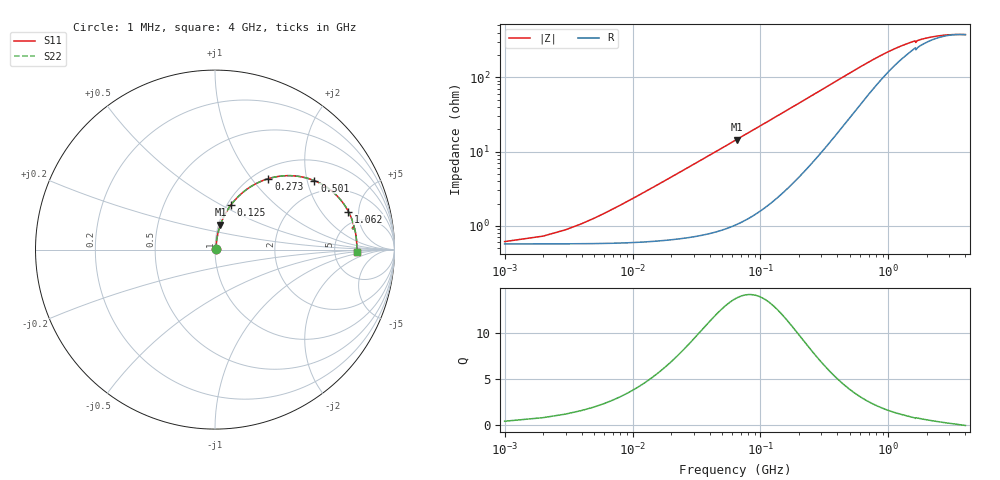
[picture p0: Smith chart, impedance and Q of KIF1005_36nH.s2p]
!version-2
!date-12.2020
!Series
# MHz S RI R 50
!Freq ReS11 ImS11 ReS21 ImS21 ReS12 ImS12 ReS22 ImS22
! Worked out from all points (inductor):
!   4000 points, 1 MHz to 4 GHz, reference 50 ohm
!   read as one part in series: L = 35.5 nH near 21 MHz
!   highest Q = 13.8 at 65 MHz (marker M1), where L = 35.4 nH
!   self-resonance near 3.685 GHz
!   S11 on the Smith chart (normalised r, x): 1 MHz: 1.01, +0.00; 125 MHz: 1.04, +0.56; 273 MHz: 1.16, +1.22; 501 MHz: 1.57, +2.22; 1.062 GHz: 3.63, +3.82; 4 GHz: 8.48, -0.50
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1  0.00569 0.00223  0.9943 -0.00223  0.9943 -0.00223  0.00569 0.00223
11  0.00657 0.0244  0.9934 -0.0244  0.9934 -0.0244  0.00657 0.0244
24  0.00951 0.0528  0.9905 -0.0528  0.9905 -0.0528  0.00951 0.0528
30  0.0114 0.0657  0.9886 -0.0657  0.9886 -0.0657  0.0114 0.0657
37  0.0142 0.0806  0.9858 -0.0806  0.9858 -0.0806  0.0142 0.0806
45  0.0179 0.0975  0.9821 -0.0975  0.9821 -0.0975  0.0179 0.0975
65  0.0301 0.1386  0.9699 -0.1386  0.9699 -0.1386  0.0301 0.1386
92  0.0527 0.1908  0.9473 -0.1908  0.9473 -0.1908  0.0527 0.1908
125  0.0882 0.248  0.9118 -0.248  0.9118 -0.248  0.0882 0.248
190  0.1757 0.3348  0.8243 -0.3348  0.8243 -0.3348  0.1757 0.3348
273  0.2979 0.3955  0.7021 -0.3955  0.7021 -0.3955  0.2979 0.3955
373  0.4299 0.4115  0.5701 -0.4115  0.5701 -0.4115  0.4299 0.4115
501  0.554 0.3841  0.446 -0.3841  0.446 -0.3841  0.554 0.3841
668  0.6517 0.3256  0.3483 -0.3256  0.3483 -0.3256  0.6517 0.3256
840  0.7065 0.2691  0.2935 -0.2691  0.2935 -0.2691  0.7065 0.2691
1062  0.7432 0.2119  0.2568 -0.2119  0.2568 -0.2119  0.7432 0.2119
1334  0.7652 0.1615  0.2348 -0.1615  0.2348 -0.1615  0.7652 0.1615
1599  0.776 0.1228  0.224 -0.1228  0.224 -0.1228  0.776 0.1228
2001  0.784 0.0881  0.216 -0.0881  0.216 -0.0881  0.784 0.0881
2667  0.7891 0.0444  0.2109 -0.0444  0.2109 -0.0444  0.7891 0.0444
3334  0.7902 0.0135  0.2098 -0.0135  0.2098 -0.0135  0.7902 0.0135
4000  0.7897 -0.011  0.2103 0.011  0.2103 0.011  0.7897 -0.011
